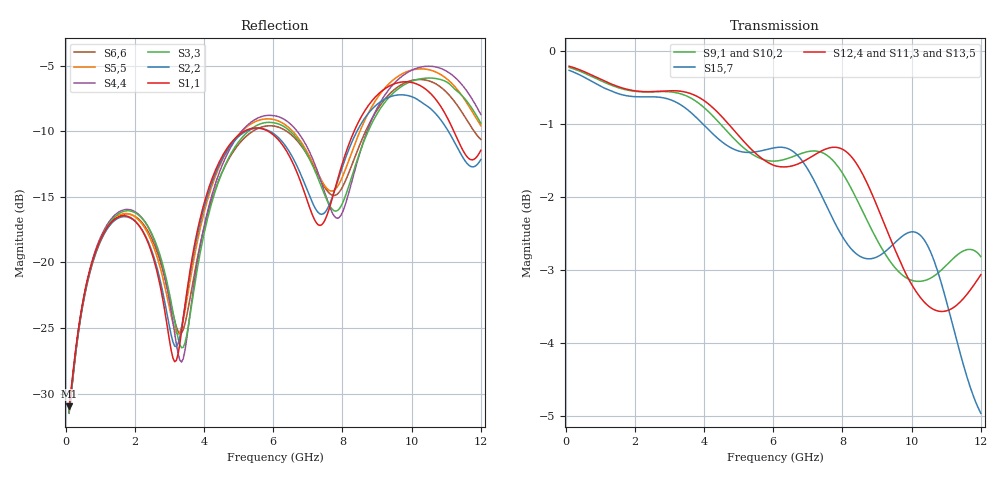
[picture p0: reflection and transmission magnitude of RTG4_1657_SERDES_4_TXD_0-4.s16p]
! RTG4 1657 S-parameter file
! Microsemi Corporation (c) 2019
!Initial ver: Jul 30, 2019
! Port::PIN_NAME::NET_NAME::S-parameter ports::PORT SIDE
! Port1:--:SERDES_4_TXD0_N_DIE::1::DIE
! Port2:--:SERDES_4_TXD0_P_DIE::2::DIE
! Port3:AW28:SERDES_4_TXD0_N_BGA::3::BGA
! Port4:AV28:SERDES_4_TXD0_P_BGA::4::BGA
! Port5:--:SERDES_4_TXD1_N_DIE::5::DIE
! Port6:--:SERDES_4_TXD1_P_DIE::6::DIE
! Port7:AU29:SERDES_4_TXD1_N_BGA::7::BGA
! Port8:AT29:SERDES_4_TXD1_P_BGA::8::BGA
! Port9:--:SERDES_4_TXD2_N_DIE::9::DIE
! Port10:--:SERDES_4_TXD2_P_DIE::10::DIE
! Port11:AU31:SERDES_4_TXD2_N_BGA::11::BGA
! Port12:AT31:SERDES_4_TXD2_P_BGA::12::BGA
! Port13:--:SERDES_4_TXD3_N_DIE::13::DIE
! Port14:--:SERDES_4_TXD3_P_DIE::14::DIE
! Port15:AU33:SERDES_4_TXD3_N_BGA::15::BGA
! Port16:AT33:SERDES_4_TXD3_P_BGA::16::BGA
!TouchstoneFormatFlag = 1
! GNDNET
! NETSLIST
! User Comments:
! Touchstone file exported from HFSS 2018.2.0
!  File:  G:/LSI/Simulation/MASUMIZU/MicroSemi/190627_KD-YB5197_Spara/YBD197_150320_NETCHANGE_SERDES_4_TXD.aedt
!  Generated:  2:00:36 ??  7 10, 2019
!  Design:  HFSSModel1
!  Project:  YBD197_150320_NETCHANGE_SERDES_4_TXD
!  Setup:  Setup1
!  Solution:  Sweep
! Terminal data exported
! Port[1] = SERDES_4_TXD0_N_DIE
! Port[2] = SERDES_4_TXD0_P_DIE
! Port[3] = SERDES_4_TXD1_N_DIE
! Port[4] = SERDES_4_TXD1_P_DIE
! Port[5] = SERDES_4_TXD2_N_DIE
! Port[6] = SERDES_4_TXD2_P_DIE
! Port[7] = SERDES_4_TXD3_N_DIE
! Port[8] = SERDES_4_TXD3_P_DIE
! Port[9] = SERDES_4_TXD0_N_BGA
! Port[10] = SERDES_4_TXD0_P_BGA
! Port[11] = SERDES_4_TXD1_N_BGA
! Port[12] = SERDES_4_TXD1_P_BGA
! Port[13] = SERDES_4_TXD2_N_BGA
! Port[14] = SERDES_4_TXD2_P_BGA
! Port[15] = SERDES_4_TXD3_N_BGA
! Port[16] = SERDES_4_TXD3_P_BGA
# GHZ S DB R 50.000000
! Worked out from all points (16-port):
!   239 points, 100 MHz to 12 GHz, reference 50 ohm
!   strongest paths, dB at 100 MHz, 3.05 GHz, 6.05 GHz, 9.05 GHz, 12 GHz:
!     S12,4: -0.2, -0.5, -1.6, -2.2, -3.1
!     S15,7: -0.3, -0.7, -1.3, -2.8, -5.0
!     S9,1: -0.2, -0.6, -1.5, -2.6, -2.8
!     S11,3: -0.2, -0.6, -1.6, -2.4, -3.3
!     S13,5: -0.2, -0.6, -1.6, -2.5, -3.1
!     S10,2: -0.2, -0.6, -1.5, -2.8, -2.8
!   lowest |S11| = -31.0 dB at 100 MHz (marker M1), VSWR 1.06, Z = 52.4 - j1.56 ohm
!   |S11| at or under -10 dB: start of sweep to 5.162 GHz; 5.849 GHz to 8.337 GHz (2.487 GHz wide, 35.1 % of centre); 11.22 GHz to end of sweep
